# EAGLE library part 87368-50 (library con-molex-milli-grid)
RECEPTACAL
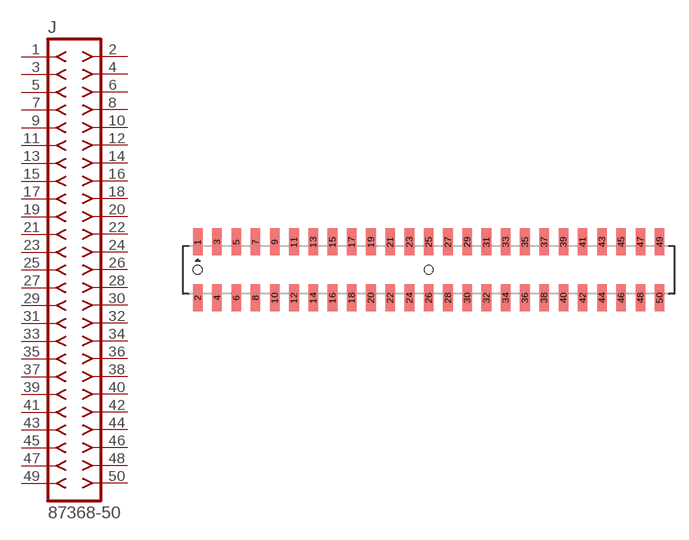
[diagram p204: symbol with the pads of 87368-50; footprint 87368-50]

Designator prefix J

## 87368-50  [87368-50]
1  1  pas
2  2  pas
3  3  pas
4  4  pas
5  5  pas
6  6  pas
7  7  pas
8  8  pas
9  9  pas
10  10  pas
11  11  pas
12  12  pas
13  13  pas
14  14  pas
15  15  pas
16  16  pas
17  17  pas
18  18  pas
19  19  pas
20  20  pas
21  21  pas
22  22  pas
23  23  pas
24  24  pas
25  25  pas
26  26  pas
27  27  pas
28  28  pas
29  29  pas
30  30  pas
31  31  pas
32  32  pas
33  33  pas
34  34  pas
35  35  pas
36  36  pas
37  37  pas
38  38  pas
39  39  pas
40  40  pas
41  41  pas
42  42  pas
43  43  pas
44  44  pas
45  45  pas
46  46  pas
47  47  pas
48  48  pas
49  49  pas
50  50  pas

## Footprint 87368-50 (pad centres in mm)
RECEPTACAL SMD Dual Row, Side Entry
smd 1 x 2.8: 1 -24,2.9; 2 -24,-2.9; 3 -22,2.9; 4 -22,-2.9; 5 -20,2.9; 6 -20,-2.9; 7 -18,2.9; 8 -18,-2.9; 9 -16,2.9; 10 -16,-2.9; 11 -14,2.9; 12 -14,-2.9; 13 -12,2.9; 14 -12,-2.9; 15 -10,2.9; 16 -10,-2.9; 17 -8,2.9; 18 -8,-2.9; 19 -6,2.9; 20 -6,-2.9; 21 -4,2.9; 22 -4,-2.9; 23 -2,2.9; 24 -2,-2.9; 25 0,2.9; 26 0,-2.9; 27 2,2.9; 28 2,-2.9; 29 4,2.9; 30 4,-2.9; 31 6,2.9; 32 6,-2.9; 33 8,2.9; 34 8,-2.9; 35 10,2.9; 36 10,-2.9; 37 12,2.9; 38 12,-2.9; 39 14,2.9; 40 14,-2.9; 41 16,2.9; 42 16,-2.9; 43 18,2.9; 44 18,-2.9; 45 20,2.9; 46 20,-2.9; 47 22,2.9; 48 22,-2.9; 49 24,2.9; 50 24,-2.9
hole 0.914 at -24,0
hole 0.914 at 0,0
